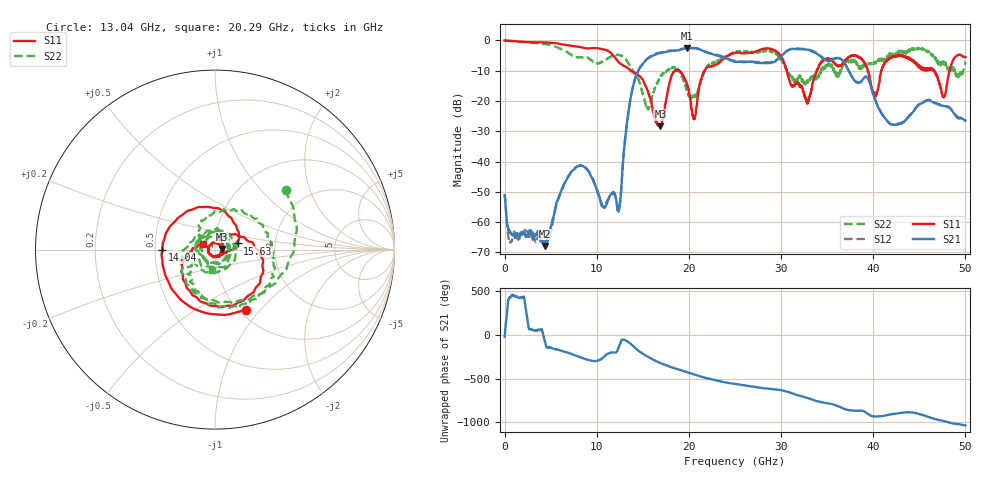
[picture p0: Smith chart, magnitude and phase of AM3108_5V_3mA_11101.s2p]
# Hz S DB R 50.0
!freq dBS11 angS11 dBS21 angS21 dBS12 angS12 dBS22 angS22
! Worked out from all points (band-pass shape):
!   1601 points, 10 MHz to 50 GHz, reference 50 ohm
!   highest |S21| = -2.49 dB at 19.82 GHz (marker M1); lowest = -67.9 dB at 4.353 GHz (marker M2)
!   |S21| within 3 dB of the highest: 15.79 GHz to 23.59 GHz (7.805 GHz wide, 39.6 % of centre); 29.92 GHz to 34.36 GHz (4.438 GHz wide, 13.8 % of centre)
!   lowest |S11| = -28.4 dB at 16.91 GHz (marker M3), VSWR 1.08, Z = 53.9 + j0.319 ohm
!   |S11| at or under -10 dB: 13.68 GHz to 18.51 GHz (4.823 GHz wide, 30 % of centre); 18.94 GHz to 21.71 GHz (2.772 GHz wide, 13.6 % of centre); 30.63 GHz to 33.85 GHz (3.225 GHz wide, 10 % of centre)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
!   |S22| runs from -22.8 to 0.0 dB; largest |S21 - S12| = 0.028
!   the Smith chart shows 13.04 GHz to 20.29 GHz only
!   S11 on the Smith chart (normalised r, x): 13.04 GHz: 1.07, -0.84; 14.04 GHz: 0.55, -0.00; 15.63 GHz: 1.28, +0.09; 20.29 GHz: 0.88, +0.06
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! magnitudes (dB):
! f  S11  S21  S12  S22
! 10 MHz  0.0  -51.2  -50.7  0.0
! 603.6 MHz  -0.1  -63.5  -66.7  -0.2
! 4.353 GHz  -0.7  -67.9  -67.3  -1.2
! 8.352 GHz  -2.3  -41.3  -41.3  -5.5
! 12.35 GHz  -7.0  -56.5  -56.2  -4.8
! 13.04 GHz  -8.5  -33.8  -33.8  -5.8
! 14.04 GHz  -10.7  -14.0  -13.9  -10.6
! 15.63 GHz  -17.7  -5.8  -5.7  -22.2
! 16.69 GHz  -28.1  -4.3  -4.1  -13.6
! 16.91 GHz  -28.4  -4.1  -4.0  -12.2
! 18.32 GHz  -10.6  -3.4  -3.3  -8.7
! 19.82 GHz  -14.7  -2.5  -2.5  -17.2
! 20.29 GHz  -22.8  -2.6  -2.5  -19.0
! 21.88 GHz  -9.1  -3.9  -3.8  -9.2
! 25 GHz  -4.1  -7.0  -6.7  -4.0
! 29.16 GHz  -3.0  -7.2  -6.9  -3.7
! 33.35 GHz  -15.9  -3.6  -3.3  -12.7
! 38 GHz  -4.8  -13.4  -13.3  -6.5
! 40.22 GHz  -18.7  -19.7  -19.5  -7.6
! 41.69 GHz  -6.1  -27.1  -27.1  -5.2
! 47.66 GHz  -18.9  -21.6  -21.6  -7.6
! 50 GHz  -5.5  -26.4  -26.7  -6.9
